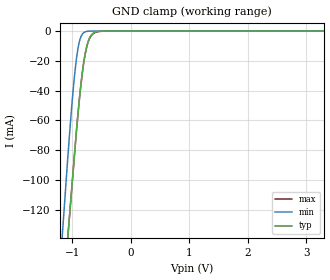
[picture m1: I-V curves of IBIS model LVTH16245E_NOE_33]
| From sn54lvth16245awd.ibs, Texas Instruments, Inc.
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[Model]   LVTH16245E_NOE_33
Model_type  Input
Vinl=0.8
Vinh=2
| variable   typ   min   max
C_comp   3.70pF   2.59pF   4.48pF
[Temperature Range]   40   -40   100
| Ambient temperature   25   -40   85
[Voltage range]   3.3   3   3.6
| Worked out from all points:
|   GND clamp passes 1 mA (typ) near -0.62 V on its own axis
[GND Clamp]
| LVTH16245E_NOE_33
|   Voltage   I(typ)   I(min)   I(max)
-5V       -2.043A    -2.266A    -2.044A
-1.175V   -186.8mA   -140.7mA   -187.5mA
-1.155V   -177.1mA   -129.6mA   -177.8mA
-1.075V   -138.3mA   -85.25mA   -139.1mA
-1.05V    -126.2mA   -72.09mA   -126.9mA
-975mV    -89.84mA   -36.15mA   -90.57mA
-925mV    -65.98mA   -18.03mA   -66.68mA
-850mV    -35.59mA   -3.758mA   -36.24mA
-775mV    -14.55mA   -465.3uA   -15.13mA
-675mV    -2.726mA   -7.638uA   -3.121mA
-510mV    -63.77uA   -5.001nA   -185.6uA
3.3V      15.85pA    3.42pA     2.911nA
